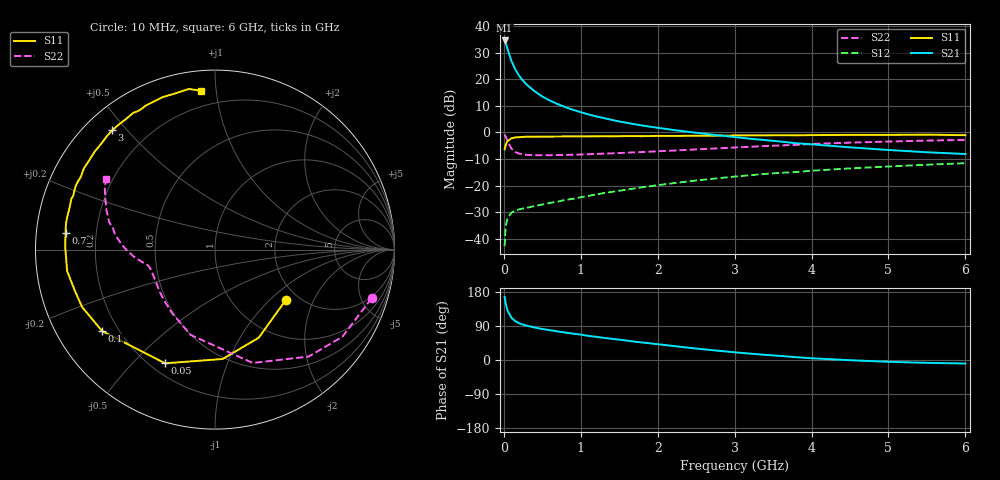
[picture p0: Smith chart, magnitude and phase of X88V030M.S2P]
! SIEMENS Small Signal Semiconductors
! BFP136W
! Si NPN RF Bipolar Junction Transistor in SOT343
! VCE = 8 V  IC = 30 mA
! Common Emitter S-Parameters:  September  1994
# GHz  S  MA  R  50
!  f  S11  S21  S12  S22
! GHz  MAG  ANG  MAG  ANG  MAG  ANG  MAG  ANG
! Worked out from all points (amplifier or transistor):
!   40 points, 10 MHz to 6 GHz, reference 50 ohm
!   highest |S21| = 34.6 dB at 10 MHz (marker M1)
!   |S21| within 3 dB of that: start of sweep to 45.39 MHz
!   unconditionally stable (mu >= 1): 891.6 MHz to 2.86 GHz
!   at 200 MHz: K = 0.41, MSG = 25.1 dB, |S12| = -28.9 dB
!   at 1.5 GHz: K = 1.12, MAG = 10.9 dB, |S12| = -21.9 dB
!   at 6 GHz: K = 0.96, MSG = 1.7 dB, |S12| = -11.5 dB
!   S11 on the Smith chart (normalised r, x): 10 MHz: 1.72, -1.26; 50 MHz: 0.26, -0.62; 100 MHz: 0.14, -0.32; 700 MHz: 0.09, +0.06; 3 GHz: 0.08, +0.46; 6 GHz: 0.11, +0.91
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0.01  0.4842 -35.3  53.4 166.7  0.0073 75.0  0.9136 -17.3
0.02  0.5481 -63.6  49.16 154.6  0.0136 66.7  0.8598 -34.4
0.03  0.6109 -86.0  45.13 144.5  0.0189 58.7  0.792 -48.8
0.05  0.692 -113.7  35.85 129.5  0.0251 44.7  0.6656 -71.6
0.1  0.7756 -144.2  21.77 111.0  0.0311 32.8  0.4944 -105.9
0.15  0.8069 -156.7  15.21 102.3  0.034 29.9  0.427 -124.2
0.2  0.8139 -163.8  11.54 96.9  0.0359 29.0  0.3999 -135.5
0.25  0.8226 -168.4  9.35 93.2  0.0373 29.0  0.3868 -142.9
0.3  0.8325 -171.8  7.85 90.4  0.0384 29.8  0.3786 -148.1
0.4  0.8309 -177.0  5.928 85.7  0.0414 32.3  0.3734 -154.8
0.5  0.8345 179.2  4.736 81.8  0.0443 34.8  0.3725 -159.1
0.6  0.8355 176.5  3.947 78.6  0.0474 37.5  0.3733 -161.6
0.7  0.8377 173.5  3.404 75.3  0.0502 39.9  0.3757 -163.4
0.9  0.8431 169.2  2.657 69.5  0.0568 43.5  0.3811 -166.1
1.1  0.8431 164.5  2.174 63.6  0.0643 46.3  0.3899 -167.6
1.5  0.8494 157.4  1.606 53.7  0.0804 50.1  0.4096 -170.1
2.2  0.8595 144.8  1.113 37.1  0.1111 50.6  0.4559 -175.3
3  0.8779 130.8  0.82 20.3  0.148 46.9  0.5209 176.9
3.2  0.8792 127.3  0.761 16.8  0.1569 45.4  0.5368 174.6
4.5  0.8982 108.9  0.524 -0.5  0.2109 35.6  0.6428 160.1
5.5  0.9066 99.2  0.424 -7.5  0.2472 27.3  0.7029 150.9
6  0.8883 94.9  0.393 -9.3  0.2646 22.9  0.7237 147.0
